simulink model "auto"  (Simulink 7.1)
settings: Solver=ode45  StartTime=0.0  StopTime=5  MaxStep=0.01  RelTol=1e-3  AbsTol=1e-3
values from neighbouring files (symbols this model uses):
  f = 2250    [auto_param.m]    (also in auto_param_opt.m = 4500; basic_control_1.m = 0.2; cf_primer4_11.m = y(nt); cf_primer4_11_1.m = y(nt))
  k1 = 7500    [auto_param.m]    (also in auto_param_opt.m = 15000)
  k2 = 150000    [auto_param.m]    (also in auto_param_opt.m)
  m = 500    [auto_param.m]    (also in auto_param_opt.m)
  y10 = 0.05    [auto_param.m]    (also in auto_param_opt.m)

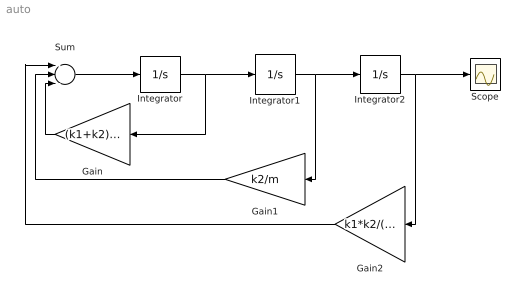
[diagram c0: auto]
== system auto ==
  Gain : Gain  Orientation=left  Gain=(k1+k2)/f  ParameterDataType=sfix(16)  ParameterScaling=2^0  OutDataType=sfix(16)  OutScaling=2^0
  Gain1 : Gain  Orientation=left  Gain=k2/m  ParameterDataType=sfix(16)  ParameterScaling=2^0  OutDataType=sfix(16)  OutScaling=2^0
  Gain2 : Gain  Orientation=left  Gain=k1*k2/(m*f)  ParameterDataType=sfix(16)  ParameterScaling=2^0  OutDataType=sfix(16)  OutScaling=2^0
  Integrator : Integrator
  Integrator1 : Integrator
  Integrator2 : Integrator  InitialCondition=-y10
  Scope : Scope
  Sum : Sum  Inputs=---  OutDataType=sfix(16)  OutScaling=2^0
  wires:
  Sum/1 -> Integrator/1
  Integrator/1 -> Integrator1/1, Gain/1
  Gain/1 -> Sum/3
  Gain1/1 -> Sum/2
  Gain2/1 -> Sum/1
  Integrator2/1 -> Gain2/1, Scope/1
  Integrator1/1 -> Gain1/1, Integrator2/1
